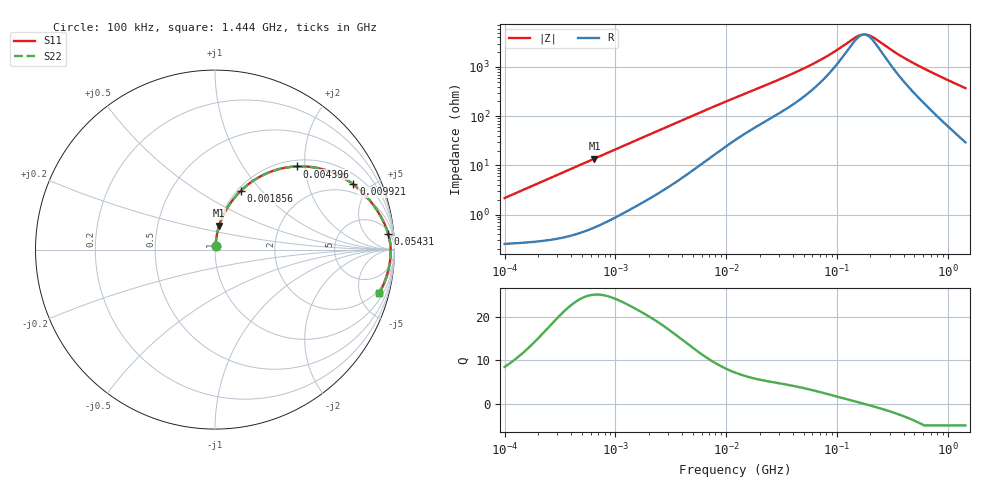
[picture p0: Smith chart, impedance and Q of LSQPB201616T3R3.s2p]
! LSQPB201616T3R3  S-PARAMETER MODEL  ( General Type )
! Model Generated by TAIYO YUDEN Corporation (http://www.ty-top.com)
! Version 2.0
! TAIYO YUDEN Control No. 100810NC14SB-FKC
! Copyright(c) 2008 TAIYO YUDEN CO.,LTD. All Rights Reserved.
! Product Description (link to TY-COMPAS)
! https://ds.yuden.co.jp/TYCOMPAS/or/detail?pn=LSQPB201616T3R3M&u=M
! Products Name : Inductors
! Characteristics :
!  Inductance : 3.3 uH , SRF(min) : 140 MHz , DC Resistance(max) : 0.286 Ohm
!  Rated Current : Saturation :740 mA , Temp Rise : 680 mA (40 degC)
!  Case Size : 2.0 x 1.6 / 0.079 x 0.063 [mm/inch] , Thickness : 1.6 / 0.063 [mm/inch]
!  (Conditions: Temperature = 25 degC , DC Bias Current/Voltage = 0A / 0V)
! External Node Assignments :
!  1  o---GGG---o  2
! GND o---------o GND
! Frequency Range : 0.1MHz  -  1443.872596MHz  [ 402 STEP ]
# MHz S RI R 50
! Freq[MHz].  S11 Real  S11 Imag  S21 Real  S21 Imag  S12 Real  S12 Imag  S22 Real  S22 Imag
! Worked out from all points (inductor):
!   401 points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, 100 kHz to 1.444 GHz, reference 50 ohm
!   read as one part in series: L = 3.43 uH near 104.9 kHz
!   highest Q = 25.2 at 647.3 kHz (marker M1), where L = 3.39 uH
!   self-resonance near 175.4 MHz
!   S11 on the Smith chart (normalised r, x): 100 kHz: 1.01, +0.04; 1.856 MHz: 1.04, +0.78; 4.396 MHz: 1.13, +1.81; 9.921 MHz: 1.48, +3.94; 54.31 MHz: 7, +20; 1.444 GHz: 1.59, -7.41
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0.1  0.003 0.0215  0.997 -0.0215  0.997 -0.0215  0.003 0.0215
0.242525  0.00567 0.0516  0.9943 -0.0516  0.9943 -0.0516  0.00567 0.0516
0.497418  0.0154 0.1042  0.9846 -0.1042  0.9846 -0.1042  0.0154 0.1042
0.647304  0.0238 0.134  0.9762 -0.134  0.9762 -0.134  0.0238 0.134
1.177819  0.0671 0.2298  0.9329 -0.2298  0.9329 -0.2298  0.0671 0.2298
1.856335  0.1433 0.327  0.8567 -0.327  0.8567 -0.327  0.1433 0.327
2.474242  0.2224 0.39  0.7776 -0.39  0.7776 -0.39  0.2224 0.39
4.395557  0.4542 0.4635  0.5458 -0.4635  0.5458 -0.4635  0.4542 0.4635
6.295007  0.6129 0.444  0.3871 -0.444  0.3871 -0.444  0.6129 0.444
9.921421  0.7707 0.3634  0.2293 -0.3634  0.2293 -0.3634  0.7707 0.3634
12.01613  0.8178 0.3229  0.1822 -0.3229  0.1822 -0.3229  0.8178 0.3229
22.93679  0.9147 0.2002  0.0853 -0.2002  0.0853 -0.2002  0.9147 0.2002
54.3113  0.965 0.0885  0.035 -0.0885  0.035 -0.0885  0.965 0.0885
59.77031  0.9676 0.0792  0.0324 -0.0792  0.0324 -0.0792  0.9676 0.0792
89.79776  0.9748 0.0449  0.0252 -0.0449  0.0252 -0.0449  0.9748 0.0449
144.9579  0.9782 0.0121  0.0218 -0.0121  0.0218 -0.0121  0.9782 0.0121
167.3535  0.9786 0.00297  0.0214 -0.00297  0.0214 -0.00297  0.9786 0.00297
184.1748  0.9787 -0.00308  0.0213 0.00308  0.0213 0.00308  0.9787 -0.00308
202.6868  0.9787 -0.00917  0.0213 0.00917  0.0213 0.00917  0.9787 -0.00917
297.308  0.9778 -0.0349  0.0222 0.0349  0.0222 0.0349  0.9778 -0.0349
581.2643  0.97 -0.0946  0.03 0.0946  0.03 0.0946  0.97 -0.0946
1443.873  0.916 -0.2405  0.084 0.2405  0.084 0.2405  0.916 -0.2405
